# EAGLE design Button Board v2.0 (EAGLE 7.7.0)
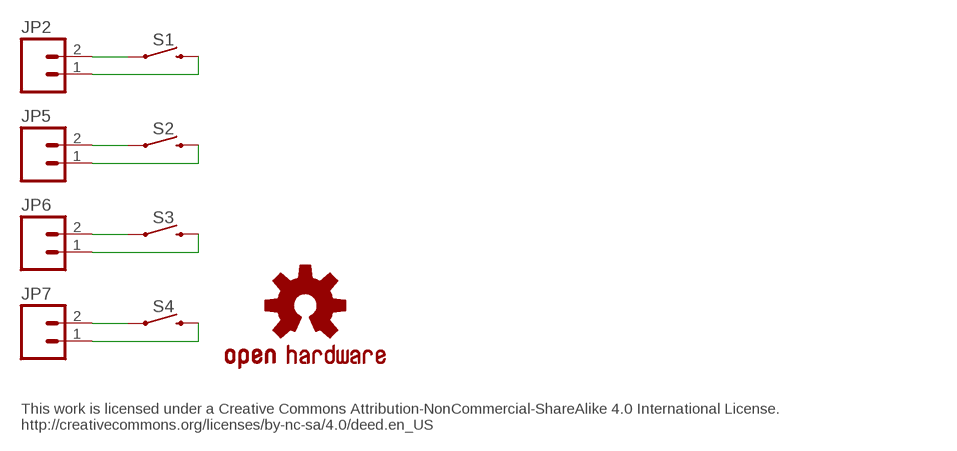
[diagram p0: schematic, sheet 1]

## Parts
JP2  M02PTH  [1X02]
JP5  M02PTH  [1X02]
JP6  M02PTH  [1X02]
JP7  M02PTH  [1X02]
S1  MOMENTARY-SWITCH-SPST-PTH-12MM  [TACTILE_SWITCH_PTH_12MM]
S2  MOMENTARY-SWITCH-SPST-PTH-12MM  [TACTILE_SWITCH_PTH_12MM]
S3  MOMENTARY-SWITCH-SPST-PTH-12MM  [TACTILE_SWITCH_PTH_12MM]
S4  MOMENTARY-SWITCH-SPST-PTH-12MM  [TACTILE_SWITCH_PTH_12MM]
U$7  OSHW-LOGOS  [OSHW-LOGO-S]

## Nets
N$1: JP2.2 S1.1
N$2: JP2.1 S1.3
N$3: JP5.2 S2.1
N$4: JP5.1 S2.3
N$5: JP6.2 S3.1
N$6: JP6.1 S3.3
N$7: JP7.2 S4.1
N$8: JP7.1 S4.3

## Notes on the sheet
- This work is licensed under a Creative Commons Attribution-NonCommercial-ShareAlike 4.0 International License.
  http://creativecommons.org/licenses/by-nc-sa/4.0/deed.en_US

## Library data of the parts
JP2 JP5-JP7 = SparkFun-Connectors:M02: Standard 2-pin 0.1" header. Use with
S1-S4 = SparkFun-Switches:MOMENTARY-SWITCH-SPST: Momentary Switch (Pushbutton) - SPST; PROD_ID: SWCH-09185; SF_SKU: COM-09190
U$7 = SparkFun:OSHW-LOGO: Open Source Hardware Logo This logo indicates the piece of hardware it is found on incorporates a OSHW license and/or adheres to the definition of open source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

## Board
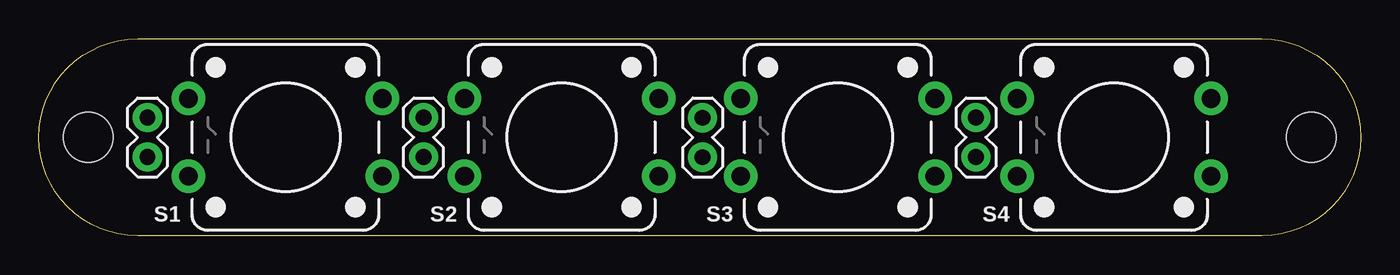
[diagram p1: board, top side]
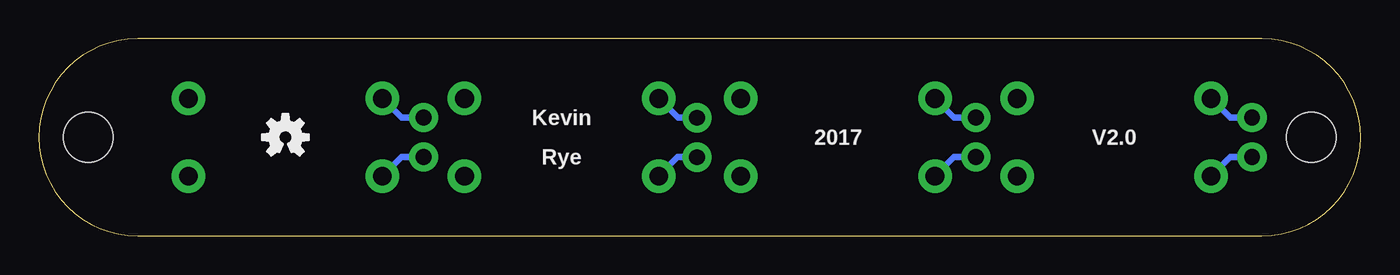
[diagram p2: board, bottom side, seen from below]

Size 85.09 x 12.7 mm. Coordinates in mm from the lower left corner, seen from the top.
Outline: 6.35,12.7 78.74,12.7 arc-180 78.74,0 6.35,0 arc-180 6.35,12.7
Copper layers (1*16): Top 0.0356mm / dielectric 1.5011mm / Bottom 0.0356mm
Design rules "LaenPCBOrder": minimum track width 6mil, minimum drill 13mil, track to track 6mil, track to pad 6mil, pad to pad 6mil, via to via 6mil, smd to smd 6mil, copper to edge 15mil, drill to drill 6mil, minimum pad ring 7mil, minimum via ring 7mil, stop-mask expansion 3mil, vias tented up to drill 0mil, thermal gap 10mil
Holes 3.2 mm at 3.17,6.35 81.92,6.35

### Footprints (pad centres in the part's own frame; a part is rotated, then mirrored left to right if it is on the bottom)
1X02 = drill 1.016 pad 1.88: 1 0,0; 2 2.54,0
TACTILE_SWITCH_PTH_12MM = drill 1.2 pad 2.159: 1 6.25,-2.5; 2 -6.25,-2.5; 3 6.25,2.5; 4 -6.25,2.5

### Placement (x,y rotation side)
JP2  6.99,5.08 90 top
JP5  24.77,5.08 90 top
JP6  42.73,5.07 90 top
JP7  60.33,5.08 90 top
S1  15.88,6.35 180 top
S2  33.66,6.35 180 top
S3  51.44,6.35 180 top
S4  69.22,6.35 180 top
U$7  69.22,6.35 0 bottom

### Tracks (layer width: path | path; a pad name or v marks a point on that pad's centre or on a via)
N$1
  Bottom 0.406: JP2.2 8.39,7.62 S1.1
N$2
  Bottom 0.406: JP2.1 8.39,5.08 S1.3
N$3
  Bottom 0.406: JP5.2 26.18,7.62 S2.1
N$4
  Bottom 0.406: JP5.1 26.18,5.08 S2.3
N$5
  Bottom 0.406: JP6.2 43.95,7.61 S3.1
N$6
  Bottom 0.406: JP6.1 43.97,5.07 S3.3
N$7
  Bottom 0.406: JP7.2 61.73,7.62 S4.1
N$8
  Bottom 0.406: JP7.1 61.73,5.08 S4.3

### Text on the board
Unrouted: This work is licensed under a Creative Commons Attribution-NonCommercial-ShareAlike 4.0 International License. / http://creativecommons.org/licenses/by-nc-sa/4.0/deed.en_US
bNames: Kevin | V2.0 | 2017 | Rye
